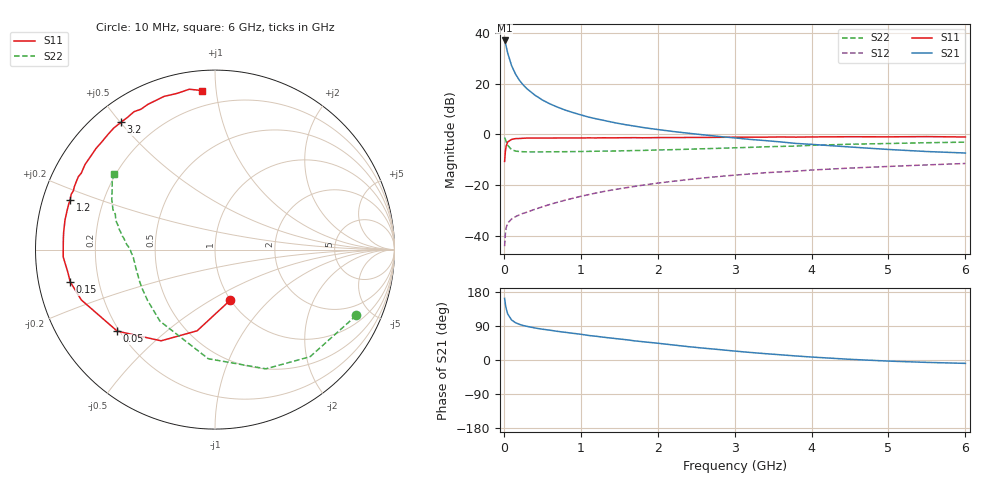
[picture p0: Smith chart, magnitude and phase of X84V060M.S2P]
! SIEMENS Small Signal Semiconductors
! BFP136W
! Si NPN RF Bipolar Junction Transistor in SOT343
! VCE = 4 V  IC = 60 mA
! Common Emitter S-Parameters:  September  1994
# GHz  S  MA  R  50
!  f  S11  S21  S12  S22
! GHz  MAG  ANG  MAG  ANG  MAG  ANG  MAG  ANG
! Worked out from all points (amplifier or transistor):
!   40 points, 10 MHz to 6 GHz, reference 50 ohm
!   highest |S21| = 37.0 dB at 10 MHz (marker M1)
!   |S21| within 3 dB of that: start of sweep to 35.37 MHz
!   unconditionally stable (mu >= 1): 647.7 MHz to 2.865 GHz
!   at 200 MHz: K = 0.58, MSG = 26.6 dB, |S12| = -31.7 dB
!   at 1.5 GHz: K = 1.10, MAG = 10.9 dB, |S12| = -21.4 dB
!   at 6 GHz: K = 0.96, MSG = 2.1 dB, |S12| = -11.5 dB
!   S11 on the Smith chart (normalised r, x): 10 MHz: 0.99, -0.61; 50 MHz: 0.19, -0.35; 150 MHz: 0.10, -0.11; 1.2 GHz: 0.08, +0.16; 3.2 GHz: 0.08, +0.50; 6 GHz: 0.11, +0.92
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0.01  0.2946 -73.4  70.75 162.6  0.0063 73.0  0.8683 -25.0
0.02  0.4632 -102.4  62.61 147.6  0.011 60.6  0.798 -48.4
0.03  0.5904 -120.6  54.35 136.3  0.0145 51.3  0.7221 -66.9
0.05  0.7094 -140.2  40.11 121.6  0.0179 40.2  0.6093 -93.5
0.1  0.7961 -159.4  22.75 105.7  0.0216 34.3  0.503 -127.6
0.15  0.8262 -167.4  15.59 98.6  0.0239 34.7  0.4704 -143.1
0.2  0.8305 -171.8  11.75 94.3  0.026 35.9  0.4602 -151.7
0.25  0.8396 -175.1  9.485 91.1  0.0279 38.4  0.456 -157.2
0.3  0.8466 -177.2  7.939 88.8  0.0294 40.4  0.4529 -161.0
0.4  0.8458 178.6  5.983 84.7  0.0334 44.4  0.4525 -165.9
0.5  0.8471 175.7  4.77 81.3  0.0375 47.6  0.453 -169.1
0.6  0.8488 173.4  3.981 78.6  0.0419 50.3  0.4539 -171.2
0.7  0.8498 170.8  3.432 75.5  0.0462 52.7  0.4555 -172.6
0.9  0.8515 167.0  2.687 70.4  0.0554 54.8  0.4586 -175.3
1.1  0.8536 162.7  2.195 64.8  0.0651 56.5  0.4633 -176.9
1.2  0.853 161.2  2.028 62.6  0.0702 57.0  0.4664 -177.7
1.7  0.863 151.9  1.454 50.5  0.0945 56.6  0.4806 178.5
2.2  0.8657 143.5  1.142 39.7  0.1194 54.0  0.5006 175.0
3.2  0.8817 126.5  0.797 20.0  0.1662 45.7  0.5555 166.2
4.5  0.8994 108.4  0.565 1.8  0.2173 34.0  0.64 154.0
5.5  0.9049 99.1  0.46 -6.3  0.2509 26.2  0.6861 146.6
6  0.889 94.7  0.43 -8.9  0.2676 21.9  0.7035 143.4
